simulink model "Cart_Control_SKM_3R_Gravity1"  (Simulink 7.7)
settings: Solver=FixedStepDiscrete  SolverMode=SingleTasking  StartTime=0  StopTime=6  FixedStep=dt  RelTol=1e-3  SampleTimeConstraint=Specified
InitFcn:
  | % Sampling Times %
  | dt0=0.001; dt1=0.01; samples=10;
  | D2R=pi/180;
undefined symbols (not defined in the file or in its folder): DiscIntNeverNeededParam, Volts
libraries: simulink_extras x4, simulink x4, speedgoatlib_IO311 x3, speedgoatlib x2, xpclib x1

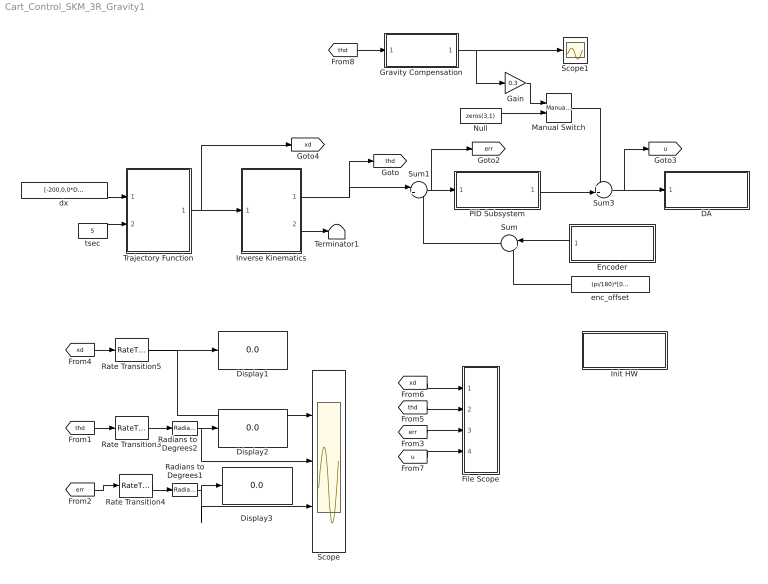
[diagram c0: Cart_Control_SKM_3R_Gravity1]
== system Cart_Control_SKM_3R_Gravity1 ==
  DA : Subsystem  TreatAsAtomicUnit=on
  Display1 : Display
  Display2 : Display
  Display3 : Display
  Encoder : Subsystem  TreatAsAtomicUnit=on
  File Scope : Subsystem
  Gain : Gain  Gain=0.3
  Gravity Compensation : Stateflow chart  TreatAsAtomicUnit=on
  Init HW : Subsystem  TreatAsAtomicUnit=on
  Inverse Kinematics : Stateflow chart  TreatAsAtomicUnit=on
  Manual Switch : simulink/Signal Routing/Manual Switch  SystemSampleTime=-1  sw=1  action=0  varsize=off
  Null : Constant  Value=zeros(3,1)
  PID Subsystem : Subsystem  TreatAsAtomicUnit=on
  Radians to Degrees1 : simulink_extras/Transformations/Radians to Degrees  SystemSampleTime=-1
  Radians to Degrees2 : simulink_extras/Transformations/Radians to Degrees  SystemSampleTime=-1
  Rate Transition3 : RateTransition  OutPortSampleTime=dt1
  Rate Transition4 : RateTransition  OutPortSampleTime=dt1
  Rate Transition5 : RateTransition  OutPortSampleTime=dt1
  Scope : Scope  NumInputPorts=3
  Scope1 : Scope
  Sum : Sum  Inputs=|++
  Sum1 : Sum  Inputs=|+-
  Sum3 : Sum  Inputs=++|
  Terminator1 : Terminator
  Trajectory Function : Stateflow chart  TreatAsAtomicUnit=on
  dx : Constant  Value=[-200,0,0*D2R]'  SampleTime=dt0
  enc_offset : Constant  Value=(pi/180)*[0,90,0]'
  tsec : Constant  Value=5  SampleTime=dt0
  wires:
  Sum1/1 -> PID Subsystem/1(In1), [err]
  PID Subsystem/1(Out1) -> Sum3/2
  Encoder/1(Out1) -> Sum/1
  enc_offset/1 -> Sum/2
  Sum/1 -> Sum1/2
  [xd] -> File Scope/1(xd)
  [thd] -> File Scope/2(thd)
  [err] -> File Scope/3(err)
  [u] -> File Scope/4(u)
  dx/1 -> Trajectory Function/1(dx)
  tsec/1 -> Trajectory Function/2(tsec)
  Trajectory Function/1(xd) -> [xd], Inverse Kinematics/1(xd)
  Inverse Kinematics/1(thd) -> Sum1/1, [thd]
  [thd] -> Rate Transition3/1
  [err] -> Rate Transition4/1
  [xd] -> Rate Transition5/1
  Rate Transition5/1 -> Display1/1, Scope/1
  Rate Transition3/1 -> Radians to Degrees2/1
  Rate Transition4/1 -> Radians to Degrees1/1
  Radians to Degrees2/1 -> Display2/1, Scope/2
  Radians to Degrees1/1 -> Display3/1, Scope/3
  Inverse Kinematics/2(w_index) -> Terminator1/1
  Manual Switch/1 -> Sum3/1
  Null/1 -> Manual Switch/2
  [thd] -> Gravity Compensation/1(thd)
  Gravity Compensation/1(out) -> Scope1/1, Gain/1
  Sum3/1 -> DA/1(In1), [u]
  Gain/1 -> Manual Switch/1

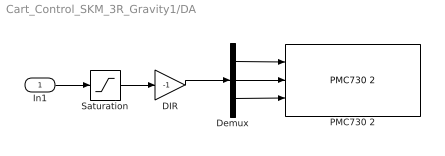
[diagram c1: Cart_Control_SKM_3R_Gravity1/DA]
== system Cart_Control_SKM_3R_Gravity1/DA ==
  In1 : Inport
  DIR : Gain  Gain=-1
  Demux : Demux  Outputs=3
  PMC730 2 : speedgoatlib/IO101/PMC730 2  id=1  channel=[1,2,3]  reset=[1,1,1]  initValue=[0,0,0]  ts=dt0  pciSlot=-1
  Saturation : Saturate  UpperLimit=10  LowerLimit=-10
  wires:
  In1/1 -> Saturation/1
  Saturation/1 -> DIR/1
  DIR/1 -> Demux/1
  Demux/1 -> PMC730 2/1
  Demux/2 -> PMC730 2/2
  Demux/3 -> PMC730 2/3

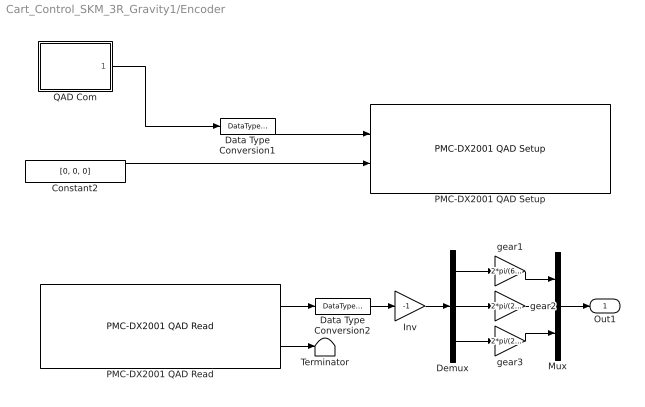
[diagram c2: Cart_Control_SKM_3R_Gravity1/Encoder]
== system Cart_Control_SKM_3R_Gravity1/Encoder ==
  Constant2 : Constant  Value=[0, 0, 0]  OutDataTypeStr=Inherit: Inherit via back propagation
  Data Type Conversion1 : DataTypeConversion  OutDataTypeStr=uint8
  Data Type Conversion2 : DataTypeConversion  OutDataTypeStr=double
  Demux : Demux  Outputs=3
  Inv : Gain  Gain=-1
  Mux : Mux  Inputs=3
  PMC-DX2001 QAD Read : speedgoatlib_IO311/PMC-DX2001 QAD Read  id=1  chan=[1, 2, 3]  pciSlot=-1  ts=dt0
  PMC-DX2001 QAD Setup : speedgoatlib_IO311/PMC-DX2001 QAD Setup  id=1  chan=Channel 3 setup  steps1=2000  steps2=2000  steps3=2000  quadrature1=4x  quadrature2=4x  quadrature3=4x  index1=Ignore index input  index2=Ignore index input  index3=Ignore index input  special1=Disabled (cycling counter)  special2=Disabled (cycling counter)  special3=Disabled (cycling counter)  debounce=0  pciSlot=-1  ts=dt0
  QAD Com : Stateflow chart  TreatAsAtomicUnit=on
  Terminator : Terminator
  gear1 : Gain  Gain=2*pi/(66*2000)
  gear2 : Gain  Gain=2*pi/(23*2000)
  gear3 : Gain  Gain=2*pi/(23*2000)
  Out1 : Outport
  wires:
  Constant2/1 -> PMC-DX2001 QAD Setup/2
  PMC-DX2001 QAD Read/2 -> Terminator/1
  PMC-DX2001 QAD Read/1 -> Data Type Conversion2/1
  QAD Com/1(y) -> Data Type Conversion1/1
  Data Type Conversion1/1 -> PMC-DX2001 QAD Setup/1
  Data Type Conversion2/1 -> Inv/1
  Mux/1 -> Out1/1
  Demux/1 -> gear1/1
  gear1/1 -> Mux/1
  Demux/2 -> gear2/1
  gear2/1 -> Mux/2
  Inv/1 -> Demux/1
  Demux/3 -> gear3/1
  gear3/1 -> Mux/3

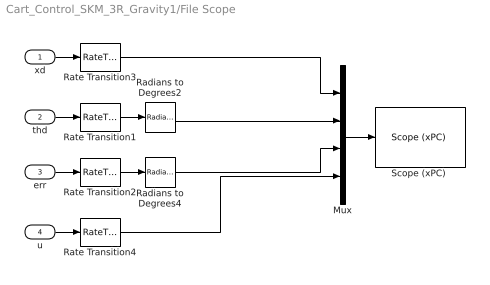
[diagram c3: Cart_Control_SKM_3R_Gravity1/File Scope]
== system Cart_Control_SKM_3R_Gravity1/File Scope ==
  xd : Inport
  thd : Inport  Port=2
  err : Inport  Port=3
  u : Inport  Port=4
  Mux : Mux
  Radians to Degrees2 : simulink_extras/Transformations/Radians to Degrees  SystemSampleTime=-1
  Radians to Degrees4 : simulink_extras/Transformations/Radians to Degrees  SystemSampleTime=-1
  Rate Transition{1..4} (4 alike) : RateTransition  OutPortSampleTime=dt1
  "Scope (xPC) " : xpclib/Misc./Scope (xPC)   SystemSampleTime=-1  scopeno=1  scopetype=File  autostart=on  viewmode=Graphical redraw  formatstr='%15.6f'  grid=on  ylimits=[0,0]  nosamples=100  noprepostsamples=0  interleave=1  triggermode=FreeRun  triggersignal=1  triggerlevel=0.0  triggerslope=Either  triggerscope=1  triggersample=0  filename=step2.dat  mode=Lazy  writesize=512  autorestart=on  dynamicfilemode=off  maxwritefilesize=512*1024^2
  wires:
  Radians to Degrees2/1 -> Mux/2
  Radians to Degrees4/1 -> Mux/3
  Rate Transition1/1 -> Radians to Degrees2/1
  Rate Transition2/1 -> Radians to Degrees4/1
  thd/1 -> Rate Transition1/1
  err/1 -> Rate Transition2/1
  Rate Transition3/1 -> Mux/1
  xd/1 -> Rate Transition3/1
  u/1 -> Rate Transition4/1
  Mux/1 -> "Scope (xPC) "/1
  Rate Transition4/1 -> Mux/4

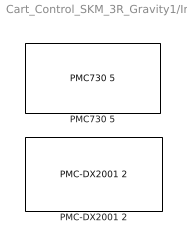
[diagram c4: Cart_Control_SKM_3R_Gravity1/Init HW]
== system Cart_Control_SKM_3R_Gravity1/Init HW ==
  PMC-DX2001 2 : speedgoatlib_IO311/PMC-DX2001 2  id=1  fpga1=IO311_3PWM_3CAP_3QAD_INT.fpga  fpga2=PWM_Triangle_DX501.fpga  fpga3=PWM_Triangle_DX501.fpga  fpga4=PWM_Triangle_DX501.fpga  fpga5=PWM_Triangle_DX501.fpga  fpga6=PWM_Triangle_DX501.fpga  fpga7=PWM_Triangle_DX501.fpga  fpga8=PWM_Triangle_DX501.fpga  fpga9=PWM_Triangle_DX501.fpga  fpga10=PWM_Triangle_DX501.fpga  group=Module setup  pciSlot=-1  lowerDirection=[ones(1,5), zeros(1, 7), ones(1, 1), ones(1, 3)]  lowerReset=[1]  lowerValue=[0]  upperDirection=[ones(1, 8), zeros(1, 8)]  upperReset=[1]  upperValue=[0]
  PMC730 5 : speedgoatlib/IO101/PMC730 5  id=1  group=Analog output setup  pciSlot=-1  adStartChannel=1  adNumChannel=1  adCoupling=Single-ended  adRange=-10 .. 10 Volts  adAcqMode=Standard  daChannel=[1,2, 3]  daReset=[1,1, 1]  daInitValue=[0,0,0]  diChannel=[1]  diDebounce=[0]  doChannel=[1]  doReset=[1]  doInitValue=[0]

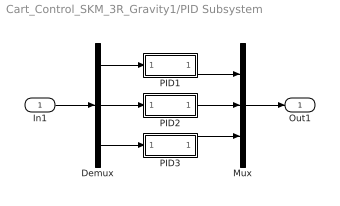
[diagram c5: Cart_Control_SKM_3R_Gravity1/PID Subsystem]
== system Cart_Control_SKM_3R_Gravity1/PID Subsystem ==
  In1 : Inport
  Demux : Demux  Outputs=3
  Mux : Mux  Inputs=3
  PID1 : Subsystem
  PID2 : Subsystem
  PID3 : Subsystem
  Out1 : Outport
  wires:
  In1/1 -> Demux/1
  Demux/1 -> PID1/1(In1)
  PID1/1(Out1) -> Mux/1
  Demux/2 -> PID2/1(In1)
  PID2/1(Out1) -> Mux/2
  Mux/1 -> Out1/1
  Demux/3 -> PID3/1(In1)
  PID3/1(Out1) -> Mux/3

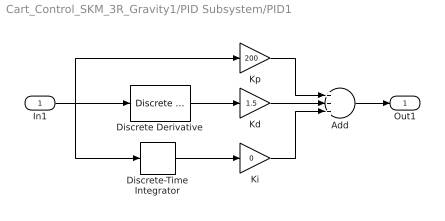
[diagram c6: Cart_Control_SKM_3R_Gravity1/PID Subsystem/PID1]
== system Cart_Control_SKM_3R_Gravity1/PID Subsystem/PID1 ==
  In1 : Inport
  Add : Sum  Inputs=+++
  Discrete Derivative : simulink/Discrete/Discrete Derivative  SystemSampleTime=-1  gainval=1.0  ICPrevScaledInput=0.0  OutMin=[]  OutMax=[]  OutDataType=fixdt(1, 16)  OutScaling=2^-10  DoSatur=off
  Discrete-Time Integrator : DiscreteIntegrator  SampleTime=dt0  ICPrevOutput=DiscIntNeverNeededParam  ICPrevScaledInput=DiscIntNeverNeededParam
  Kd : Gain  Gain=1.5
  Ki : Gain  Gain=0
  Kp : Gain  Gain=200
  Out1 : Outport
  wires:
  Discrete-Time Integrator/1 -> Ki/1
  Kp/1 -> Add/1
  Kd/1 -> Add/2
  Ki/1 -> Add/3
  Discrete Derivative/1 -> Kd/1
  Add/1 -> Out1/1
  In1/1 -> Kp/1, Discrete Derivative/1, Discrete-Time Integrator/1

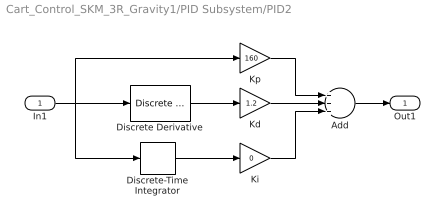
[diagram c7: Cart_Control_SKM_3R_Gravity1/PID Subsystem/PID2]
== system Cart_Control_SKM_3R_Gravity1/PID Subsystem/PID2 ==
  In1 : Inport
  Add : Sum  Inputs=+++
  Discrete Derivative : simulink/Discrete/Discrete Derivative  SystemSampleTime=-1  gainval=1.0  ICPrevScaledInput=0.0  OutMin=[]  OutMax=[]  OutDataType=fixdt(1, 16)  OutScaling=2^-10  DoSatur=off
  Discrete-Time Integrator : DiscreteIntegrator  SampleTime=dt0  ICPrevOutput=DiscIntNeverNeededParam  ICPrevScaledInput=DiscIntNeverNeededParam
  Kd : Gain  Gain=1.2
  Ki : Gain  Gain=0
  Kp : Gain  Gain=160
  Out1 : Outport
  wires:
  Discrete-Time Integrator/1 -> Ki/1
  Kp/1 -> Add/1
  Kd/1 -> Add/2
  Ki/1 -> Add/3
  Discrete Derivative/1 -> Kd/1
  Add/1 -> Out1/1
  In1/1 -> Kp/1, Discrete Derivative/1, Discrete-Time Integrator/1

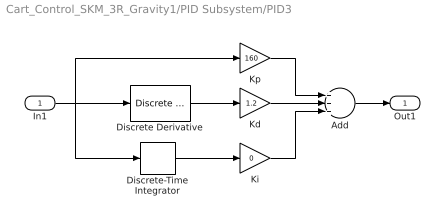
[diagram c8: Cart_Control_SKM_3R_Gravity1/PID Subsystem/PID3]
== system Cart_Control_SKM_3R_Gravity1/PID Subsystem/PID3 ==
  In1 : Inport
  Add : Sum  Inputs=+++
  Discrete Derivative : simulink/Discrete/Discrete Derivative  SystemSampleTime=-1  gainval=1.0  ICPrevScaledInput=0.0  OutMin=[]  OutMax=[]  OutDataType=fixdt(1, 16)  OutScaling=2^-10  DoSatur=off
  Discrete-Time Integrator : DiscreteIntegrator  SampleTime=dt0  ICPrevOutput=DiscIntNeverNeededParam  ICPrevScaledInput=DiscIntNeverNeededParam
  Kd : Gain  Gain=1.2
  Ki : Gain  Gain=0
  Kp : Gain  Gain=160
  Out1 : Outport
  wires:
  Discrete-Time Integrator/1 -> Ki/1
  Kp/1 -> Add/1
  Kd/1 -> Add/2
  Ki/1 -> Add/3
  Discrete Derivative/1 -> Kd/1
  Add/1 -> Out1/1
  In1/1 -> Kp/1, Discrete Derivative/1, Discrete-Time Integrator/1

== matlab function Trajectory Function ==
function xd = fcn(dx, tsec)

persistent index xd_p

MAX_CH=3;       % 3 Actuators %
dt=0.001;       % Step time is 10 msec %
a1=100; a2=70; a3=50;

% Initializing Variables %
if isempty(index), index=0; end
if isempty(xd_p), xd_p=zeros(MAX_CH,1); end
xd=zeros(MAX_CH,1);
x0=[a1,a2+a3, pi/2]';

tout=index*dt;
if index<(tsec/dt)
    [c] = coeff_3rd(x0, zeros(MAX_CH,1), x0+dx, zeros(MAX_CH,1), tsec);
    for ch=1:MAX_CH
        xd(ch,1)=c(ch,1)+c(ch,2)*tout+c(ch,3)*tout^2+c(ch,4)*tout^3;    
    end
    xd_p=xd;
else
    xd=xd_p;
end
index=index+1;

function [c] = coeff_3rd(sp, sv, ep, ev, tsec)
MAX_CH=3;
c=zeros(MAX_CH,4);
for ch=1:MAX_CH
    c(ch,1)=sp(ch,1);
    c(ch,2)=sv(ch,1);
    c(ch,3)=(3.0*(ep(ch,1)-sp(ch,1))-(2.0*sv(ch,1)+ev(ch,1))*tsec)/(tsec*tsec);
    c(ch,4)=(-2.0*(ep(ch,1)-sp(ch,1))+(sv(ch,1)+ev(ch,1))*tsec)/(tsec*tsec*tsec);
end

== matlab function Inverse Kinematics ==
function [thd,w_index]  = fcn(xd)

persistent index thd_p

% Initializing Variables %
if isempty(index), index=0; end
if isempty(thd_p), thd_p=(pi/180)*[0,90,0]'; end

w_index=1;  % In workspace %
a1=100; a2=70; a3=50;

qx=xd(1,1); qy=xd(2,1); phi=xd(3,1);

% (1) Calculate th2 %
px=qx-a3*cos(phi); py=qy-a3*sin(phi);
kapha=(px^2+py^2-a1^2-a2^2)/(2*a1*a2);
if abs(kapha)>1
    w_index=-1;  % Out of Workspace %
    kapha=1;
end
th2=+acos(kapha); % Elbow Down %
%th2=-acos(kapha); % Elbow Up %
 
% (2) Calculate th1 %
delta=a1^2+a2^2+2*a1*a2*cos(th2);
cth1=(px*(a1+a2*cos(th2))+py*a2*sin(th2))/delta;
sth1=(-px*a2*sin(th2)+py*(a1+a2*cos(th2)))/delta;
th1=atan2(sth1, cth1);
if th1<0, th1=th1+2*pi; end % 0<th<360 %

% (3) Calcuate th3 %
th3=phi-(th1+th2);

% (3) Check Joint Limits %
if th1<0 || th1>pi, w_index=-1; end
if th2<pi/6 || th2>5*pi/6, w_index=-1; end

% Result %
if w_index==1
    thd=[th1, th2, th3]';
else
    thd=thd_p;
end

% Save the current value %
thd_p=thd;

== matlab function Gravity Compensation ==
function out = fcn(thd)

MM2M=0.001;

th1=thd(1,1); th2=thd(2,1); th3=thd(3,1);
tau=zeros(3,1);
out=zeros(3,1);

% Robot Parameters %
m1=0.363; a1=MM2M*100; ac1=MM2M*87.74;
m2=0.292; a2=MM2M*70; ac2=MM2M*62.65;
m3=0.050; ac3=MM2M*18.60; %a3=MM2M*50;
g=-9.81;    % Gravity Direction -Y axis %

tau(1,1)=g*(m1*ac1*cos(th1)+m2*(a1*cos(th1)+ac2*cos(th1+th2))...
    +m3*(a1*cos(th1)+a2*cos(th1+th2))+ac3*cos(th1+th2+th3));
tau(2,1)=m2*g*ac2*cos(th1+th2)+m3*g*(a2*cos(th1+th2)+ac3*cos(th1+th2+th3));
tau(3,1)=m3*g*ac3*cos(th1+th2+th3);

% Motor Torque Constant 10[V]/Max Torque[Nm] %
ratio=66/23;

out(1,1)=tau(1,1);
out(2,1)=ratio*tau(2,1);
out(3,1)=ratio*tau(3,1);

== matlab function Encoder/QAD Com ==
function y = fcn()

persistent index

if isempty(index), index=0; end

if index==0
    y=[1,1,1];      %  Reset %
else
    y = [0,0,0];
end

index=index+1;
